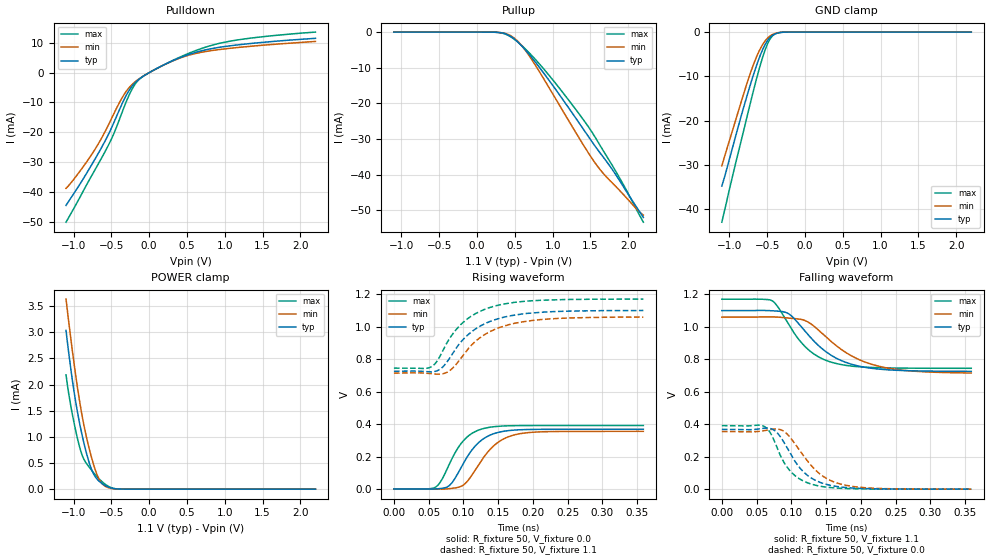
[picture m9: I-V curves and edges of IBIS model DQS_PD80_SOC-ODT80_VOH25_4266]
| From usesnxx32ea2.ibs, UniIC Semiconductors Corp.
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| DQS_PD80_SOC-ODT80_VOH25_4266
| (80 Ohm Pulldown, 80 Ohm System ODT Setting, VOH=VDDQ/2.5, 3200-4266Mbps)
[Model]   DQS_PD80_SOC-ODT80_VOH25_4266
Model_type   I/O
Vinl = 160.000mV
Vinh = 280.000mV
Vmeas = 220.000mV
Vref = 0.0mV
Cref = 0.0pF
Rref = 80.000Ohm
|   typ   min   max
|C_comp   0.849pF   0.799pF   0.899pF
C_comp_pullup   0.4245pF   0.3995pF   0.4495pF
C_comp_pulldown   0.4245pF   0.3995pF   0.4495pF
| Note: C_comp changes when the ODT circuit is enabled.
[Model Spec]
| Input threshold voltage corners
Vinl   0.1600V   0.1520V   0.1740V
Vinh   0.2800V   0.2720V   0.2940V
| Measurement voltage corners
Vmeas   0.2200V   0.2120V   0.2340V
| Timing spec test load voltage corners
Vref   0.0000V   0.0000V   0.0000V
| Dynamic Overshoot Parameters from LPDDR4 Specification
D_overshoot_ampl_h   0.30   NA   NA
D_overshoot_ampl_l   0.30   NA   NA
D_overshoot_area_h   0.1n   NA   NA
D_overshoot_area_l   0.1n   NA   NA
[Voltage Range]   1.1000V   1.0600V   1.1700V
[Pullup Reference]   1.1000V   1.0600V   1.1700V
| Junction Temperature (Ambient temp is 35C typ 95C min -40C max)
[Temperature Range]   50.0   110.0   -40.0
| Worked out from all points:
|   slope of the pulldown table from 0 to 0.165 V, typ, clamps not added: 73.8 ohm
|   slope of the pullup table from 0 to 0.165 V, typ, clamps not added: 17.5 kohm
|   GND clamp passes 1 mA (typ) near -0.45 V on its own axis
|   POWER clamp passes 1 mA (typ) near -0.88 V on its own axis
|   rising waveform, R_fixture 50, V_fixture 0.0: 20-80 % time 35.1ps typ, 38.9ps min, 32ps max; typ from 0.001 V to 0.368 V
|   falling waveform, R_fixture 50, V_fixture 1.1: 20-80 % time 58ps typ, 69ps min, 47.3ps max; typ from 1.1 V to 0.726 V
|   rising waveform, R_fixture 50, V_fixture 1.1: 20-80 % time 54.9ps typ, 56.7ps min, 51.7ps max; typ from 0.726 V to 1.1 V
|   falling waveform, R_fixture 50, V_fixture 0.0: 20-80 % time 38.3ps typ, 44.3ps min, 32.9ps max; typ from 0.368 V to 0.001 V
[Pulldown]
|   Voltage   I(typ)   I(min)   I(max)
-1.1V     -44.48mA   -38.75mA   -50.1mA
-921.8mV  -37.58mA   -33.22mA   -42.04mA
-720.5mV  -29.14mA   -25.86mA   -32.73mA
-489.5mV  -18.03mA   -14.96mA   -21.71mA
-314.6mV  -8.178mA   -6.693mA   -10.48mA
-212.3mV  -4.114mA   -3.666mA   -4.927mA
-110mV    -1.768mA   -1.705mA   -1.812mA
381.7mV   4.717mA    4.613mA    4.889mA
589.6mV   6.577mA    6.251mA    7.117mA
883.3mV   8.277mA    7.574mA    9.509mA
1.368V    9.806mA    8.868mA    11.62mA
2.2V      11.48mA    10.44mA    13.57mA
[GND Clamp]
|   Voltage   I(typ)   I(min)   I(max)
-1.1V     -34.75mA   -30.2mA    -42.92mA
-1.05V    -31.86mA   -27.33mA   -39.27mA
-948.2mV  -25.44mA   -21.62mA   -31.8mA
-789.8mV  -15.73mA   -12.78mA   -20.73mA
-664.4mV  -8.74mA    -6.576mA   -12.08mA
-595.1mV  -5.401mA   -3.898mA   -7.695mA
-525.8mV  -2.768mA   -1.974mA   -3.966mA
-473mV    -1.422mA   -1.031mA   -1.89mA
-416.9mV  -600.9uA   -440.5uA   -665.8uA
-357.5mV  -192.8uA   -144.2uA   -174uA
-248.6mV  -12.2uA    -10.93uA   -7.146uA
2.2V      0A         0A         0A
[Pullup]
|   Voltage   I(typ)   I(min)   I(max)
-1.1V     4.106uA    7.431uA    1.361uA
259.6mV   -60.57uA   -59.49uA   -61.51uA
388.3mV   -576.6uA   -480.7uA   -687.8uA
500.5mV   -2.04mA    -1.831mA   -2.142mA
619.3mV   -4.529mA   -4.567mA   -4.328mA
754.6mV   -7.982mA   -8.738mA   -7.279mA
1.042V    -16.16mA   -18.8mA    -14.47mA
1.448V    -28.55mA   -33.09mA   -25.83mA
1.662V    -34.9mA    -39.5mA    -33.05mA
1.788V    -38.54mA   -42.33mA   -37.4mA
1.943V    -43.63mA   -45.77mA   -43.12mA
2.2V      -52.05mA   -51.39mA   -53.39mA
[POWER Clamp]
|   Voltage   I(typ)   I(min)   I(max)
-1.1V     3.033mA    3.633mA    2.184mA
-1.044V   2.381mA    2.967mA    1.653mA
-981.2mV  1.752mA    2.276mA    1.183mA
-911.9mV  1.201mA    1.611mA    764.5uA
-855.8mV  837.8uA    1.172mA    552.1uA
-796.4mV  521.2uA    795.3uA    427.2uA
-743.6mV  316uA      510.6uA    330.1uA
-674.3mV  169.2uA    226uA      215.1uA
-598.4mV  83.65uA    71.95uA    113.1uA
-486.2mV  16.75uA    10.13uA    20.98uA
-367.4mV  1.201uA    871.3nA    948.2nA
2.2V      0A         0A         0A
[Ramp]
|   typ   min   max
| 20% - 80%
dV/dt_r   220.51m/35.12p   212.86m/38.87p   234.61m/31.95p
dV/dt_f   224.46m/57.99p   206.41m/68.96p   255.16m/47.24p
| 25% - 75%
|dV/dt_r   183.76m/27.95p   177.38m/30.96p   195.51m/25.38p
|dV/dt_f   187.05m/46.15p   172.01m/54.89p   212.64m/37.50p
R_load = 50
[Rising Waveform]
R_fixture = 50
V_fixture = 0.0
|   Time   V(typ)   V(min)   V(max)
0s        836.2uV    685.8uV    613uV
58ps      506.9uV    -45.3uV    7.832mV
67ps      3.418mV    -439.2uV   44.62mV
77ps      13.93mV    1.482mV    127.9mV
86ps      53.46mV    5.803mV    207.8mV
102ps     173.7mV    31.95mV    306.9mV
129ps     310.1mV    194.6mV    373mV
152ps     351mV      294.2mV    387.2mV
181ps     365.2mV    340.8mV    391mV
359ps     368.4mV    355.4mV    391.6mV
[Falling Waveform]
R_fixture   = 50
V_fixture   = 1.1
V_fixture_min = 1.06
V_fixture_max = 1.17
|   Time   V(typ)   V(min)   V(max)
0s        1.1V       1.06V      1.17V
73ps      1.099V     1.061V     1.159V
96ps      1.081V     1.054V     1.016V
118ps     982.4mV    1.041V     886.3mV
137ps     893.3mV    987.8mV    820.4mV
157ps     825.9mV    911.1mV    782.9mV
191ps     764.5mV    811.4mV    756.4mV
230ps     738.2mV    753.4mV    747.8mV
284ps     728.3mV    724.8mV    745.2mV
359ps     725.9mV    716mV      744.7mV
[Rising Waveform]
R_fixture   = 50
V_fixture   = 1.1
V_fixture_min = 1.06
V_fixture_max = 1.17
|   Time   V(typ)   V(min)   V(max)
0s        725.5mV    714.2mV    744.7mV
53ps      721.5mV    710.7mV    751.4mV
62ps      728.2mV    707.5mV    787.3mV
75ps      774.9mV    716.2mV    890.4mV
89ps      864.6mV    765.3mV    979mV
107ps     951.9mV    864.6mV    1.052V
124ps     1.003V     932.4mV    1.095V
145ps     1.042V     982.9mV    1.127V
209ps     1.088V     1.043V     1.162V
359ps     1.1V       1.059V     1.17V
[Falling Waveform]
R_fixture = 50
V_fixture = 0.0
|   Time   V(typ)   V(min)   V(max)
0s        368.5mV    355.6mV    391.7mV
58ps      374.4mV    359mV      391.8mV
74ps      367mV      370.3mV    313.1mV
86ps      312.3mV    364.2mV    192.4mV
98ps      224.6mV    321.2mV    114.5mV
114ps     122.9mV    226.6mV    58.43mV
132ps     61.05mV    130.3mV    27.72mV
157ps     23.47mV    52.97mV    10.16mV
191ps     6.912mV    15.81mV    2.96mV
359ps     897.5uV    805.7uV    637uV
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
